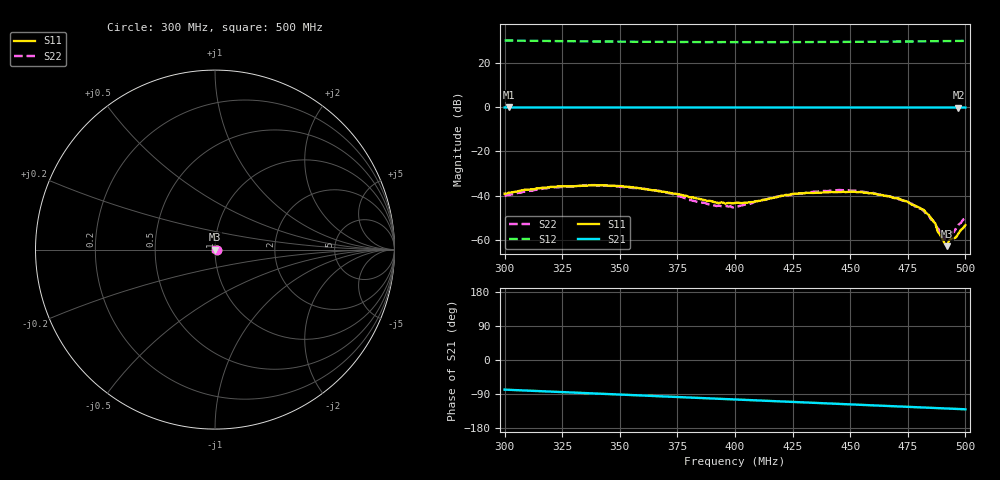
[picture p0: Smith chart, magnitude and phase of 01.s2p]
!Prosund Technologies,SP809B,SP82221046,V.03.04.C
!Date: Monday, March 31, 2025 16:26:08
!Correction: S11(C* 2-Port  )
!S21(C* 2-Port  )
!S12(C* 2-Port  )
!S22(C* 2-Port  )
!S2P File: Measurement: :
# Hz S  dB  R 50
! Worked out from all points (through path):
!   201 points, 300 MHz to 500 MHz, reference 50 ohm
!   highest |S21| = -0.06 dB at 302 MHz (marker M1); lowest = -0.1 dB at 497 MHz (marker M2)
!   group delay of S21, straight-line fit = 721 ps
!   lowest |S11| = -62.9 dB at 492 MHz (marker M3), VSWR 1.00, Z = 50.1 + j0.048 ohm
!   |S11| at or under -10 dB: start of sweep to end of sweep
!   |S22| runs from -59.7 to -35.2 dB; largest |S21 - S12| = 32
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3e8  -39.13 -11.1  -0.06 -78.2  30.30 -89.5  -40.23 -10.1
3.02e8  -38.58 -12.1  -0.06 -78.7  30.28 -89.5  -39.69 -11.2
3.34e8  -35.49 -26.2  -0.07 -87.0  29.89 -89.6  -35.45 -14.6
3.49e8  -35.63 -21.6  -0.07 -90.9  29.73 -89.5  -35.89 -12.4
3.67e8  -38.09 -12.1  -0.07 -95.6  29.63 -89.5  -37.82 -2.5
3.85e8  -41.62 -11.7  -0.08 -100.3  29.58 -89.7  -43.19 -9.9
3.93e8  -43.39 -16.5  -0.08 -102.3  29.54 -89.3  -44.50 -25.4
4e8  -43.33 -32.9  -0.08 -104.2  29.55 -89.6  -44.95 -36.7
4.19e8  -40.44 -53.6  -0.08 -109.1  29.57 -89.6  -40.30 -58.2
4.2e8  -40.13 -54.6  -0.08 -109.3  29.52 -89.7  -40.19 -57.4
4.22e8  -39.70 -56.1  -0.08 -109.9  29.58 -89.5  -39.89 -58.7
4.34e8  -38.80 -61.7  -0.08 -113.0  29.59 -89.5  -38.29 -51.9
4.53e8  -38.49 -55.0  -0.08 -117.9  29.68 -89.7  -37.88 -43.0
4.63e8  -39.69 -48.6  -0.08 -120.5  29.74 -89.3  -39.51 -36.7
4.66e8  -40.26 -46.5  -0.08 -121.3  29.81 -89.6  -40.12 -35.3
4.67e8  -40.36 -46.8  -0.08 -121.5  29.78 -89.7  -40.37 -34.5
4.69e8  -41.11 -46.1  -0.08 -122.0  29.77 -89.4  -40.88 -34.6
4.82e8  -46.52 -39.6  -0.08 -125.4  29.92 -89.4  -47.07 -16.8
4.91e8  -61.68 14.4  -0.09 -127.8  29.99 -89.5  -59.66 43.1
4.92e8  -62.92 42.2  -0.08 -128.0  30.03 -89.4  -57.46 64.6
4.97e8  -57.14 102.2  -0.09 -129.3  30.10 -89.7  -53.23 114.2
5e8  -53.33 124.5  -0.09 -130.1  30.10 -89.5  -50.37 121.7
